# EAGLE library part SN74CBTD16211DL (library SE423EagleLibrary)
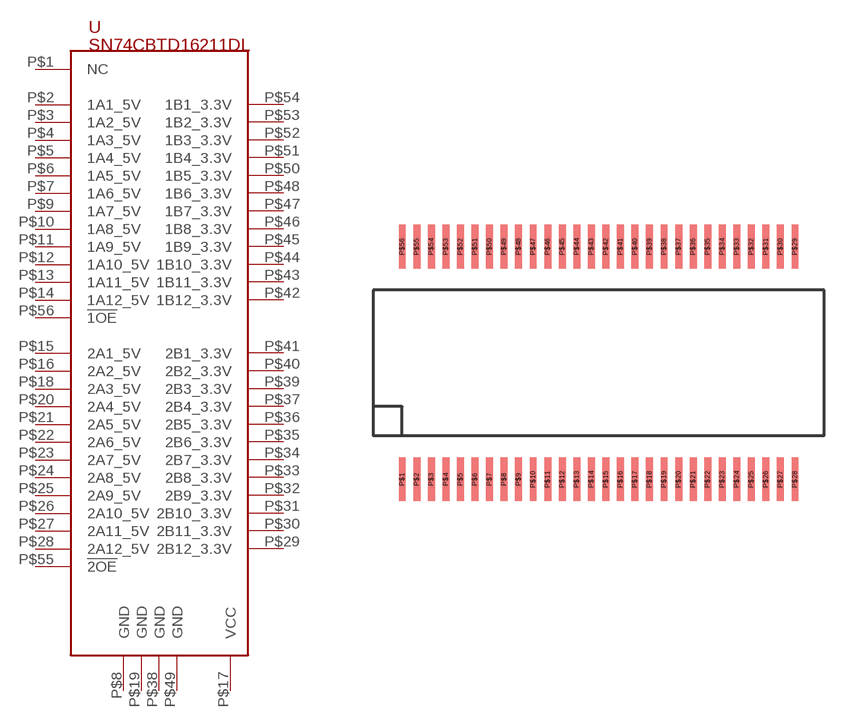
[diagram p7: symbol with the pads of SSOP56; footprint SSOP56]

Designator prefix U

## SN74CBTD16211DL  [SSOP56]
P$1  NC
P$2  1A1_5V
P$3  1A2_5V
P$4  1A3_5V
P$5  1A4_5V
P$6  1A5_5V
P$7  1A6_5V
P$8  GND
P$9  1A7_5V
P$10  1A8_5V
P$11  1A9_5V
P$12  1A10_5V
P$13  1A11_5V
P$14  1A12_5V
P$15  2A1_5V
P$16  2A2_5V
P$17  VCC
P$18  2A3_5V
P$19  GND
P$20  2A4_5V
P$21  2A5_5V
P$22  2A6_5V
P$23  2A7_5V
P$24  2A8_5V
P$25  2A9_5V
P$26  2A10_5V
P$27  2A11_5V
P$28  2A12_5V
P$29  2B12_3.3V
P$30  2B11_3.3V
P$31  2B10_3.3V
P$32  2B9_3.3V
P$33  2B8_3.3V
P$34  2B7_3.3V
P$35  2B6_3.3V
P$36  2B5_3.3V
P$37  2B4_3.3V
P$38  GND
P$39  2B3_3.3V
P$40  2B2_3.3V
P$41  2B1_3.3V
P$42  1B12_3.3V
P$43  1B11_3.3V
P$44  1B10_3.3V
P$45  1B9_3.3V
P$46  1B8_3.3V
P$47  1B7_3.3V
P$48  1B6_3.3V
P$49  GND
P$50  1B5_3.3V
P$51  1B4_3.3V
P$52  1B3_3.3V
P$53  1B2_3.3V
P$54  1B1_3.3V
P$55  !2OE
P$56  !1OE

## Footprint SSOP56 (pad centres in mm)
smd 0.305 x 1.905: P$1 0,-5.08; P$2 0.635,-5.08; P$3 1.27,-5.08; P$4 1.905,-5.08; P$5 2.54,-5.08; P$6 3.175,-5.08; P$7 3.81,-5.08; P$8 4.445,-5.08; P$9 5.08,-5.08; P$10 5.715,-5.08; P$11 6.35,-5.08; P$12 6.985,-5.08; P$13 7.62,-5.08; P$14 8.255,-5.08; P$15 8.89,-5.08; P$16 9.525,-5.08; P$17 10.16,-5.08; P$18 10.795,-5.08; P$19 11.43,-5.08; P$20 12.065,-5.08; P$21 12.7,-5.08; P$22 13.335,-5.08; P$23 13.97,-5.08; P$24 14.605,-5.08; P$25 15.24,-5.08; P$26 15.875,-5.08; P$27 16.51,-5.08; P$28 17.145,-5.08; P$29 17.145,5.08; P$30 16.51,5.08; P$31 15.875,5.08; P$32 15.24,5.08; P$33 14.605,5.08; P$34 13.97,5.08; P$35 13.335,5.08; P$36 12.7,5.08; P$37 12.065,5.08; P$38 11.43,5.08; P$39 10.795,5.08; P$40 10.16,5.08; P$41 9.525,5.08; P$42 8.89,5.08; P$43 8.255,5.08; P$44 7.62,5.08; P$45 6.985,5.08; P$46 6.35,5.08; P$47 5.715,5.08; P$48 5.08,5.08; P$49 4.445,5.08; P$50 3.81,5.08; P$51 3.175,5.08; P$52 2.54,5.08; P$53 1.905,5.08; P$54 1.27,5.08; P$55 0.635,5.08; P$56 0,5.08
